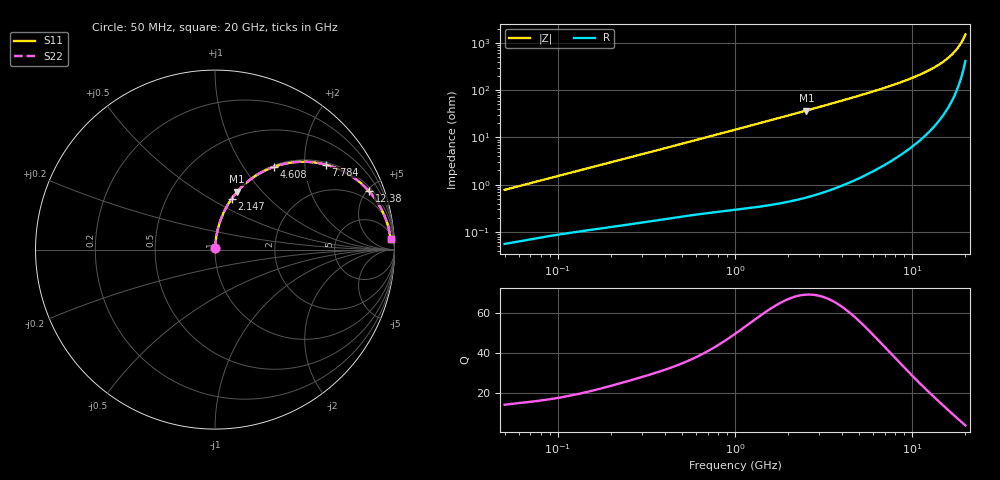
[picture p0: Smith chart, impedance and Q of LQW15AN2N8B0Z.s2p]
!Murata Part Number: LQW15AN2N8B0Z
!These Parameters are Measured in Series Mode Connection
!  o--[Z]--o
!Port1  Port2
!  o-------o
!Freq. Start=50[MHz] Stop=20[GHz], 401[Steps]
# Hz S RI R 50
!Freq.(Hz) S11(Real) S11(Imag) S21(Real) S21(Imag) S12(Real) S12(Imag) S22(Real) S22(Imag)
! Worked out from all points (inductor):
!   401 points, 50 MHz to 20 GHz, reference 50 ohm
!   read as one part in series: L = 2.45 nH near 51.52 MHz
!   highest Q = 69.1 at 2.531 GHz (marker M1), where L = 2.33 nH
!   S11 on the Smith chart (normalised r, x): 50 MHz: 1.00, +0.02; 2.147 GHz: 1.01, +0.63; 4.608 GHz: 1.02, +1.39; 7.784 GHz: 1.07, +2.56; 12.38 GHz: 1.25, +5.19; 20 GHz: 9, +29
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5e7  0.000619 0.00775  0.9994 -0.00775  0.9994 -0.00775  0.000619 0.00775
1.364002e8  0.00146 0.0204  0.9985 -0.0204  0.9985 -0.0204  0.00146 0.0204
3.721004e8  0.00476 0.0543  0.9952 -0.0543  0.9952 -0.0543  0.00476 0.0543
6.285508e8  0.0107 0.0905  0.9893 -0.0905  0.9893 -0.0905  0.0107 0.0905
1e9  0.0234 0.1414  0.9766 -0.1414  0.9766 -0.1414  0.0234 0.1414
1.521052e9  0.0497 0.2092  0.9503 -0.2092  0.9503 -0.2092  0.0497 0.2092
2.146657e9  0.0926 0.2826  0.9074 -0.2826  0.9074 -0.2826  0.0926 0.2826
2.531158e9  0.1241 0.3225  0.8759 -0.3225  0.8759 -0.3225  0.1241 0.3225
2.728004e9  0.1414 0.3413  0.8586 -0.3413  0.8586 -0.3413  0.1414 0.3413
3.572216e9  0.2223 0.4082  0.7777 -0.4082  0.7777 -0.4082  0.2223 0.4082
4.608136e9  0.3283 0.4612  0.6717 -0.4612  0.6717 -0.4612  0.3283 0.4612
5.944466e9  0.4613 0.4885  0.5387 -0.4885  0.5387 -0.4885  0.4613 0.4885
7.442007e9  0.5918 0.4793  0.4082 -0.4793  0.4082 -0.4793  0.5918 0.4793
7.784049e9  0.6182 0.473  0.3818 -0.473  0.3818 -0.473  0.6182 0.473
1.004137e10  0.7607 0.4094  0.2393 -0.4094  0.2393 -0.4094  0.7607 0.4094
1.238412e10  0.859 0.3244  0.141 -0.3244  0.141 -0.3244  0.859 0.3244
1.460232e10  0.918 0.2419  0.082 -0.2419  0.082 -0.2419  0.918 0.2419
1.646126e10  0.9493 0.1757  0.0507 -0.1757  0.0507 -0.1757  0.9493 0.1757
1.800918e10  0.9661 0.1237  0.0339 -0.1237  0.0339 -0.1237  0.9661 0.1237
1.855685e10  0.9704 0.1061  0.0296 -0.1061  0.0296 -0.1061  0.9704 0.1061
1.940974e10  0.9755 0.0793  0.0245 -0.0793  0.0245 -0.0793  0.9755 0.0793
2e10  0.9781 0.0614  0.0219 -0.0614  0.0219 -0.0614  0.9781 0.0614
